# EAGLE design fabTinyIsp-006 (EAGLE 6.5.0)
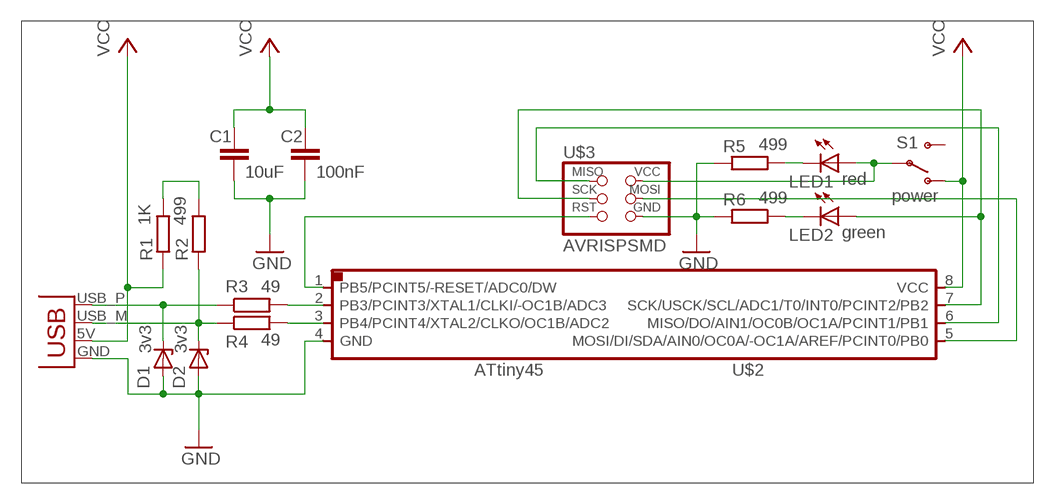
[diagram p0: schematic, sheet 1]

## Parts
C1  10uF  C-EUC1206  [C1206]
C2  100nF  C-EUC1206  [C1206]
D1  3v3  ZENER_DIODESOD123  [SOD123]
D2  3v3  ZENER_DIODESOD123  [SOD123]
LED1  red  LEDSMT1206  [1206]
LED2  green  LEDSMT1206  [1206]
R1  1K  R-EU_R1206  [R1206]
R2  499  R-EU_R1206  [R1206]
R3  49  R-EU_R1206  [R1206]
R4  49  R-EU_R1206  [R1206]
R5  499  R-EU_R1206  [R1206]
R6  499  R-EU_R1206  [R1206]
S1  power  SWITCH-SPSTSMD2  [SWITCH-SPDT-SMD]
U$1  USBPCB  [USB-A-PCB]
U$2  ATTINY45SI  [SOIC8]
U$3  AVRISPSMD  [2X03SMD]

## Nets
GND: C1.2 C2.2 D1.ANODE D2.ANODE R5.2 R6.2 U$1.GND U$2.4(GND) U$3.6(GND)
N$1: R1.2 R2.2
N$2: R4.2 U$2.3(PB4/PCINT4/XTAL2/CLKO/OC1B/ADC2)
N$3: D1.CATHODE R3.1 U$1.USB_P(D+)
N$4: R3.2 U$2.2(PB3/PCINT3/XTAL1/CLKI/-OC1B/ADC3)
N$5: D2.CATHODE R2.1 R4.1 U$1.USB_M(D-)
N$6: U$2.1(PB5/PCINT5/-RESET/ADC0/DW) U$3.5(RST)
N$9: U$2.5(MOSI/DI/SDA/AIN0/OC0A/-OC1A/AREF/PCINT0/PB0) U$3.4(MOSI)
N$10: U$2.6(MISO/DO/AIN1/OC0B/OC1A/PCINT1/PB1) U$3.1(MISO)
N$11: LED2.A U$2.7(SCK/USCK/SCL/ADC1/T0/INT0/PCINT2/PB2) U$3.3(SCK)
N$12: LED1.A S1.2(P) U$3.2(VCC)
N$13: LED2.C R6.1
N$14: LED1.C R5.1
VCC: C1.1 C2.1 R1.1 S1.1(O) U$1.5V(VBUS) U$2.8(VCC)
Unconnected: S1.3(S)

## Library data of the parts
C1 C2 = rcl:C-EU: CAPACITOR, European symbol
D1 D2 = 01_fab:ZENER_DIODE: zener diode
LED1 LED2 = led:LED: LED
R1-R6 = resistor:R-EU_: RESISTOR, European symbol
S1 = SparkFun:SWITCH-SPST: SPST Switch Simple slide switch. Spark Fun Electronics SKU : COM-00102
U$1 = SparkFun:USB: USB Connectors USB-B-PTH is fully proven SKU : PRT-00139 USB-miniB is fully proven SKU : PRT-00587 USB-A-PCB is untested. USB-A-H is throughly reviewed, but untested. Spark Fun Electronics SKU : PRT-00437 USB-B-SMT is throughly reviewed, but untested. Needs silkscreen touching up. USB-A-S has not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
U$2 = 01_fab:ATTINY45
U$3 = 01_fab:AVRISP

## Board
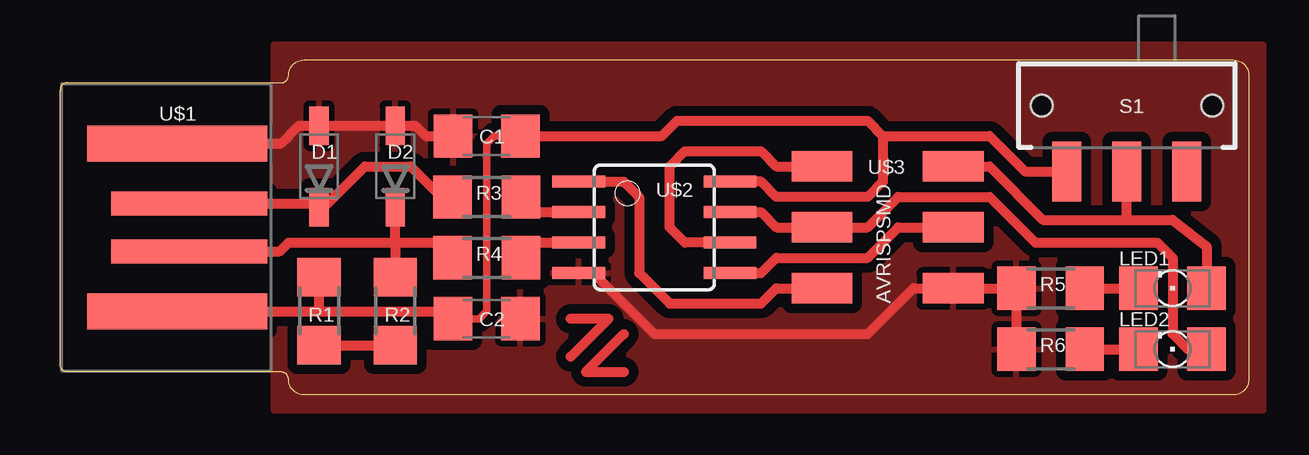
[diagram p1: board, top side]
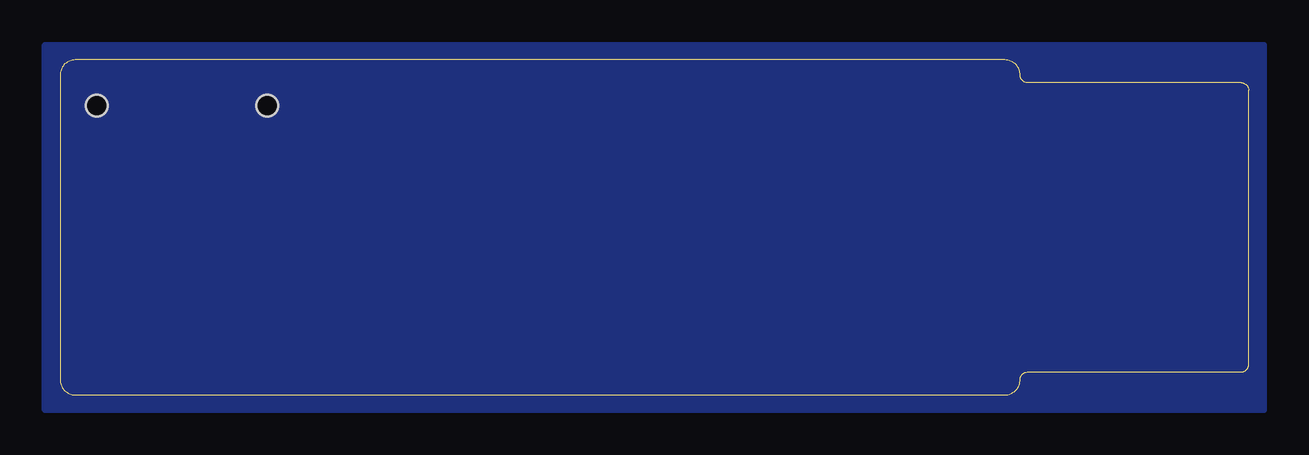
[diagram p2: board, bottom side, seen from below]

Size 49.53 x 13.97 mm. Coordinates in mm from the lower left corner, seen from the top.
Outline: 9.21,13.02 arc90 9.53,13.34 arc-90 10.16,13.97 48.9,13.97 arc-90 49.53,13.34 49.53,0.64 arc-90 48.9,0 10.16,0 arc-90 9.53,0.64 arc90 9.21,0.95 0.32,0.95 arc-90 0,1.27 0,12.7 arc-90 0.32,13.02 9.21,13.02
Copper layers (1*16): Top 0.035mm / dielectric 1.5mm / Bottom 0.035mm
Design rules "default *": minimum track width 10mil, minimum drill 24mil, track to track 16mil, track to pad 16mil, pad to pad 16mil, via to via 16mil, smd to smd 8mil, copper to edge 0mil, drill to drill 8mil, minimum pad ring 10mil, minimum via ring 8mil, stop-mask expansion 4mil, vias tented up to drill 0mil, thermal gap 10mil

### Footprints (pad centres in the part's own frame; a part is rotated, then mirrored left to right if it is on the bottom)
C1206 = smd 1.6 x 1.8: 1 -1.4,0; 2 1.4,0
SOD123 = smd 1.6 x 0.8: ANODE 1.7,0; CATHODE -1.7,0
1206 = smd 1.6 x 1.803: A -1.422,0; C 1.422,0
R1206 = smd 1.6 x 1.803: 1 -1.422,0; 2 1.422,0
SWITCH-SPDT-SMD = smd 1.2 x 2.5: 1 -2.5,-2.75; 2 0,-2.75; 3 2.5,-2.75 | hole 0.9: -3.55,0; 3.55,0
USB-A-PCB = smd 7.5 x 1.5: 5V -0.2,-3.5; GND -0.2,3.5 | smd 6.5 x 1: USB_M 0.3,-1; USB_P 0.3,1
SOIC8 = smd 0.5 x 2.2: 1 -1.905,-3.154; 2 -0.645,-3.154; 3 0.625,-3.154; 4 1.895,-3.154; 5 1.905,3.154; 6 0.635,3.154; 7 -0.635,3.154; 8 -1.905,3.154
2X03SMD = smd 2.54 x 1.27: 1 -2.54,2.54; 2 2.92,2.54; 3 -2.54,0; 4 2.92,0; 5 -2.54,-2.54; 6 2.92,-2.54

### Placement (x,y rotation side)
C1  17.78,10.79 180 top
C2  17.78,3.17 0 top
D1  10.79,9.53 90 top
D2  13.97,9.53 90 top
LED1  46.35,4.45 180 top
LED2  46.35,1.91 180 top
R1  10.79,3.49 270 top
R2  13.97,3.49 270 top
R3  17.78,8.26 0 top
R4  17.78,5.71 0 top
R5  41.27,4.45 180 top
R6  41.27,1.91 180 top
S1  44.45,12.06 0 top
U$1  5.08,6.99 0 top
U$2  24.77,6.99 270 top
U$3  34.29,6.99 0 top

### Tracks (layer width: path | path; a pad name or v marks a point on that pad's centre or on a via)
GND
  Top 0.406: R6.2 R5.2 U$3.6 35.56,4.45 33.66,2.54 24.77,2.54 22.21,5.09 U$2.4 | U$1.GND 9.21,10.48 9.96,11.22 D1.ANODE D2.ANODE 14.81,11.22 15.24,10.79 C1.2
  pour Top: 8.89,-0.64 50.16,-0.64 50.16,14.61 8.89,14.61
N$1
  Top 0.406: R1.2 R2.2
N$2
  Top 0.406: U$2.3 19.85,6.36 R4.2
N$3
  Top 0.406: U$1.USB_P 10.63,7.99 D1.CATHODE 11,7.83 12.7,9.53 14.61,9.53 15.88,8.26 R3.1
N$4
  Top 0.406: U$2.2 19.83,7.63 R3.2
N$5
  Top 0.406: 13.97,6.35 D2.CATHODE | U$1.USB_M 9.16,5.99 9.53,6.35 13.97,6.35 | 13.97,6.35 R2.1 | 13.97,6.35 15.72,6.35 R4.1
N$6
  Top 0.406: U$2.1 23.5,8.89 24.13,8.26 24.13,5.08 25.4,3.81 29.21,3.81 29.84,4.45 U$3.5
N$9
  Top 0.406: U$2.5 29.21,5.08 29.84,5.71 33.66,5.71 34.92,6.99 U$3.4
N$10
  Top 0.406: U$2.6 26.04,6.35 25.4,6.99 25.4,9.53 26.04,10.16 29.21,10.16 29.84,9.53 U$3.1
N$11
  Top 0.406: U$2.7 29.21,7.62 29.84,6.99 U$3.3 33.66,6.99 34.92,8.26 38.73,8.26 40.64,6.35 45.72,6.35 46.35,5.71 46.35,2.54 46.99,1.91 LED2.A
N$12
  Top 0.406: 44.45,7.3 46.35,7.3 47.78,6.2 LED1.A | 44.45,7.3 S1.2 | U$3.2 38.73,9.53 40.96,7.3 44.45,7.3
N$13
  Top 0.406: R6.1 LED2.C
N$14
  Top 0.406: R5.1 LED1.C
N$15
  pour Bottom: -0.64,-0.64 50.16,-0.64 50.16,14.61 -0.64,14.61
N$16
  Top 0.406: 21.27,3.17 22.86,3.17 21.27,1.59
N$17
  Top 0.406: 23.5,2.54 21.91,0.95 23.5,0.95
VCC
  Top 0.305: C2.1 17.46,3.17 17.78,3.49 17.78,10.48 18.1,10.79 C1.1
  Top 0.406: 34.29,10.79 34.29,8.89 33.66,8.26 29.84,8.26 29.21,8.89 U$2.8 | S1.1 40.22,9.31 38.73,10.79 34.29,10.79 | 34.29,10.79 33.66,11.43 25.72,11.43 25.08,10.79 C1.1 | U$1.5V 10.79,3.48 | 10.79,3.48 R1.1 | 10.79,3.48 16.07,3.48 C2.1

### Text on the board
tDocu: FabTinyISP v0.1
